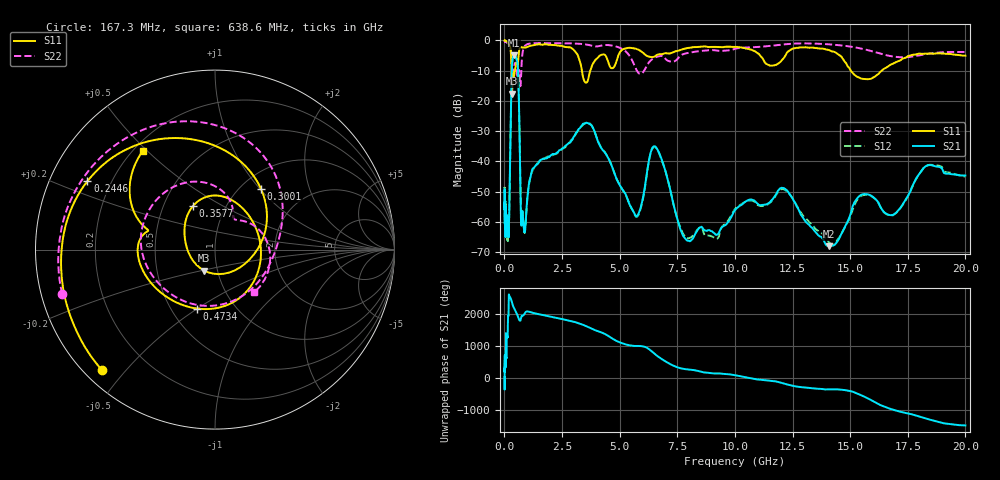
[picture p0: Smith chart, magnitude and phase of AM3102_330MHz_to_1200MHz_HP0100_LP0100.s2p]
! Date/Time: Tue, Sep 11, 2018 5:12 PM
! Network Analyzer: Agilent Technologies E8362B Rev: A.07.50.63
! Sweep from 0.010 to 20.000 GHz, 1601 Points, Sweep Type: LOG
! Power Supply: 4.949 V, 0.001 A
# Hz S DB R 50
!freq MagS11 AngS11 MagS21 AngS21 MagS12 AngS12 MagS22 AngS22
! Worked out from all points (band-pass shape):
!   1601 points, 10 MHz to 20 GHz, reference 50 ohm
!   highest |S21| = -4.87 dB at 420.4 MHz (marker M1); lowest = -68.1 dB at 14.07 GHz (marker M2)
!   |S21| within 3 dB of the highest: 334.6 MHz to 573.2 MHz (238.6 MHz wide, 52.6 % of centre)
!   lowest |S11| = -17.6 dB at 330 MHz (marker M3), VSWR 1.30, Z = 43.2 - j10.2 ohm
!   |S11| at or under -10 dB: 307.8 MHz to 457.1 MHz (149.3 MHz wide, 39 % of centre); 3.364 GHz to 3.727 GHz (363.5 MHz wide, 10.3 % of centre); 15.03 GHz to 16.37 GHz (1.347 GHz wide, 8.58 % of centre)
!   |S22| runs from -15.2 to -0.2 dB; largest |S21 - S12| = 0.0089
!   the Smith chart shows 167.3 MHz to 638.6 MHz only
!   S11 on the Smith chart (normalised r, x): 167.3 MHz: 0.05, -0.43; 244.6 MHz: 0.11, +0.25; 300.1 MHz: 1.24, +1.01; 357.7 MHz: 0.70, +0.36; 473.4 MHz: 0.67, -0.50; 638.6 MHz: 0.24, +0.49
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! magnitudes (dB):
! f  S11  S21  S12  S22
! 10 MHz  0.0  -60.5  -48.6  -0.2
! 35.55 MHz  0.0  -56.9  -60.1  -0.4
! 126.4 MHz  -0.4  -63.0  -62.0  -0.8
! 167.3 MHz  -0.7  -62.5  -64.2  -1.0
! 244.6 MHz  -1.9  -42.0  -42.2  -1.9
! 300.1 MHz  -7.5  -16.7  -16.8  -4.3
! 330 MHz  -17.6  -8.5  -8.5  -8.3
! 357.7 MHz  -11.3  -6.1  -6.2  -10.5
! 420.4 MHz  -11.8  -4.9  -4.9  -8.6
! 447.2 MHz  -10.5  -5.0  -5.0  -7.7
! 473.4 MHz  -9.3  -5.2  -5.2  -7.4
! 638.6 MHz  -3.3  -22.9  -23.0  -9.8
! 726 MHz  -2.3  -60.4  -60.0  -11.7
! 869.7 MHz  -2.3  -63.3  -63.5  -2.1
! 1.59 GHz  -1.4  -39.5  -39.5  -0.9
! 3.651 GHz  -12.3  -27.5  -27.2  -1.5
! 5.652 GHz  -2.6  -57.5  -57.7  -8.4
! 6.549 GHz  -5.2  -35.1  -35.3  -5.6
! 7.92 GHz  -2.5  -66.2  -65.5  -4.2
! 12.09 GHz  -6.1  -48.8  -49.2  -1.3
! 14.07 GHz  -3.2  -68.1  -66.7  -1.3
! 20 GHz  -5.0  -44.7  -45.1  -3.8
